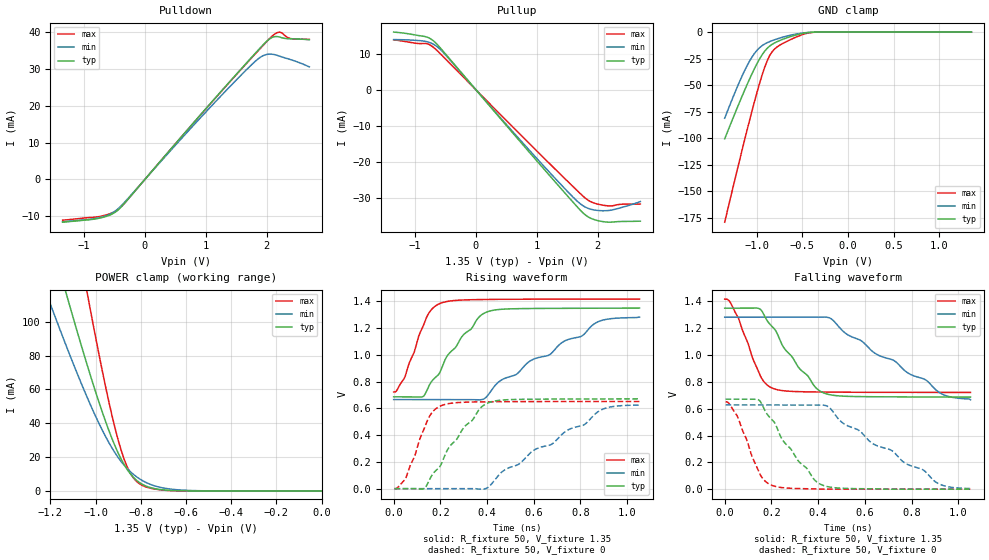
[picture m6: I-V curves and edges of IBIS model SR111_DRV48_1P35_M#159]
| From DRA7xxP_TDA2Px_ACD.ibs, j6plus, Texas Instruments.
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| Model based on original model for DDR_SEIOPB_V
|   Sub model SR111_DRV48_1P35
[model]   SR111_DRV48_1P35_M#159
|[Description]  [1.35V-I/O-X-X]
|   , ,
|[Input Load]
|[Output Drive]
|Voltage   1.35V
|Mode   I/O
Model_type   I/O
Polarity   Non-Inverting
Enable   Active-Low
Vinl =  0.585
Vinh =  0.765
Cref =  15.0000pF
Rref =  100.0000M
Vref =  0V
Vmeas =  0.675
C_comp   2p   2p   2p
[Model Spec]
Vinl   0.585   0.55125   0.61875
Vinh   0.765   0.73125   0.79875
[Receiver Thresholds]
Tslew_ac = 5n
Vth = 0.675
Vth_max = 0.709
Vth_min = 0.608
Vinh_ac = 0.175
Vinh_dc = 0.1
Vinl_ac = -0.175
Vinl_dc = -0.1
[Temperature Range]   25   125   -40
[Voltage Range]   1.35   1.2825   1.4175
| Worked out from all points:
|   slope of the pulldown table from 0 to 0.203 V, typ, clamps not added: 51.5 ohm
|   slope of the pullup table from 0 to 0.203 V, typ, clamps not added: 50.4 ohm
|   GND clamp passes 1 mA (typ) near -0.48 V on its own axis
|   POWER clamp passes 1 mA (typ) near -0.72 V on its own axis
|   rising waveform, R_fixture 50, V_fixture 1.35: 20-80 % time 170ps typ, 374ps min, 87.2ps max; typ from 0.687 V to 1.35 V
|   rising waveform, R_fixture 50, V_fixture 0: 20-80 % time 167ps typ, 368ps min, 85.2ps max; typ from 0 V to 0.671 V
|   falling waveform, R_fixture 50, V_fixture 1.35: 20-80 % time 165ps typ, 357ps min, 90.5ps max; typ from 1.35 V to 0.687 V
|   falling waveform, R_fixture 50, V_fixture 0: 20-80 % time 167ps typ, 363ps min, 86.3ps max; typ from 0.671 V to 0 V
[POWER_clamp]
-1.35V    224.4mA    165.8mA    358.5mA
-1.214V   157mA      115.5mA    250.8mA
-1.132V   117.8mA    86.59mA    187.7mA
-1.118V   111.4mA    81.92mA    177.3mA
-1.036V   74.26mA    55.16mA    116.8mA
-954.5mV  40.7mA     31.91mA    61.06mA
-900mV    22.42mA    19.79mA    30.14mA
-859.1mV  12.48mA    13.09mA    13.96mA
-804.5mV  4.85mA     7.084mA    4.132mA
-736.4mV  1.313mA    2.9mA      1.073mA
-627.3mV  101.6uA    577.3uA    45.9uA
0V        75.63nA    322.4nA    418.5nA
[Pulldown]
-1.35V    -11.61mA   -11.5mA    -11.06mA
-736.4mV  -10.48mA   -10.33mA   -10.03mA
-531.8mV  -9.35mA    -9.062mA   -9.043mA
-409.1mV  -7.817mA   -7.49mA    -7.751mA
1.145V    21.94mA    20.88mA    21.88mA
1.718V    32.55mA    30.62mA    32.41mA
1.923V    36.25mA    33.48mA    36.08mA
2.005V    37.61mA    33.98mA    37.53mA
2.086V    38.57mA    34.03mA    38.89mA
2.209V    38.7mA     33.51mA    40.04mA
2.373V    38.22mA    32.66mA    38.36mA
2.7V      37.95mA    30.56mA    38.05mA
[Pullup]
-1.35V    15.95mA    13.86mA    13.81mA
-981.8mV  15.11mA    13.66mA    12.86mA
-818.2mV  14.65mA    13.35mA    12.79mA
-736.4mV  14.02mA    12.92mA    12.23mA
-613.6mV  12.13mA    11.6mA     10.47mA
1.064V    -20.91mA   -20.19mA   -18.01mA
1.555V    -30.35mA   -29.03mA   -26.14mA
1.759V    -34.1mA    -32.12mA   -29.45mA
1.923V    -35.82mA   -33.22mA   -31.26mA
2.168V    -36.64mA   -33.43mA   -32.13mA
2.414V    -36.45mA   -32.48mA   -31.67mA
2.7V      -36.37mA   -30.94mA   -31.63mA
[GND_clamp]
-1.35V    -100.7mA   -81.27mA   -179.3mA
-1.241V   -77.31mA   -57.61mA   -140mA
-1.132V   -54.83mA   -36.31mA   -101.6mA
-1.05V    -39.08mA   -23.36mA   -74mA
-968.2mV  -25.28mA   -14.71mA   -48.34mA
-913.6mV  -18.13mA   -11.32mA   -33.52mA
-859.1mV  -13.28mA   -9.024mA   -22.35mA
-831.8mV  -11.61mA   -8.091mA   -18.64mA
-777.3mV  -9.078mA   -6.444mA   -14.07mA
-531.8mV  -1.871mA   -1.307mA   -3.441mA
-368.2mV  -88.76uA   -111.2uA   -158uA
1.35V     75.63nA    385.5nA    349.4nA
[Ramp]
dV/dt_f 0.39875542/0.16540827n 0.37093885/0.35831576n 0.41803136/90.620728p
dV/dt_r 0.40475857/0.16803272n 0.37926751/0.36987796n   0.392221/85.405985p
R_load = 50
[Rising Waveform]
R_fixture = 50
V_fixture = 1.35
V_fixture_min = 1.2825
V_fixture_max = 1.4175
0s        686.6mV    666.1mV    722.8mV
47.08ps   686mV      666.1mV    831.3mV
125.7ps   688.6mV    666mV      1.213V
156.7ps   786.2mV    666mV      1.328V
201ps     880.8mV    666.1mV    1.386V
294.6ps   1.142V     665.9mV    1.41V
407.2ps   1.326V     706.8mV    1.415V
457.4ps   1.341V     807.8mV    1.415V
869.5ps   1.349V     1.243V     1.417V
1.053ns   1.35V      1.282V     1.417V
[Rising Waveform]
R_fixture = 50
V_fixture = 0
V_fixture_min = 0
V_fixture_max = 0
3.741ps   0V         0V         0V
50.57ps   0V         0V         74.33mV
131.1ps   0V         0V         450.1mV
163ps     97.25mV    0V         566.1mV
209.8ps   207.5mV    0V         624.6mV
300.4ps   456.6mV    0V         646mV
413.4ps   647.1mV    23.89mV    649.7mV
472.4ps   663.5mV    136.6mV    650.5mV
885.1ps   670.7mV    585.7mV    651.7mV
1.056ns   671.4mV    628.3mV    651.8mV
[Falling Waveform]
R_fixture = 50
V_fixture = 1.35
V_fixture_min = 1.2825
V_fixture_max = 1.4175
0s        1.35V      1.282V     1.417V
21ps      1.35V      1.283V     1.401V
57.32ps   1.35V      1.283V     1.281V
147.1ps   1.347V     1.283V     867mV
207.4ps   1.206V     1.283V     751.2mV
316.9ps   906.9mV    1.282V     727.3mV
430.4ps   713.7mV    1.284V     724.2mV
861.2ps   687.7mV    814.3mV    721.9mV
924.6ps   687.4mV    715.3mV    721.9mV
1.053ns   686.6mV    666.1mV    721.8mV
[Falling Waveform]
R_fixture = 50
V_fixture = 0
V_fixture_min = 0
V_fixture_max = 0
3.741ps   671.4mV    628.3mV    651.8mV
55.04ps   671.5mV    628.3mV    541.1mV
143ps     667.7mV    628.3mV    142.2mV
206ps     513.1mV    628.3mV    25.98mV
312.6ps   216mV      628.2mV    4.532mV
424.4ps   26.43mV    626.4mV    0V
629.7ps   2.464mV    344.6mV    0V
714ps     0V         289.3mV    0V
911.6ps   0V         44.58mV    0V
1.056ns   0V         0V         0V
